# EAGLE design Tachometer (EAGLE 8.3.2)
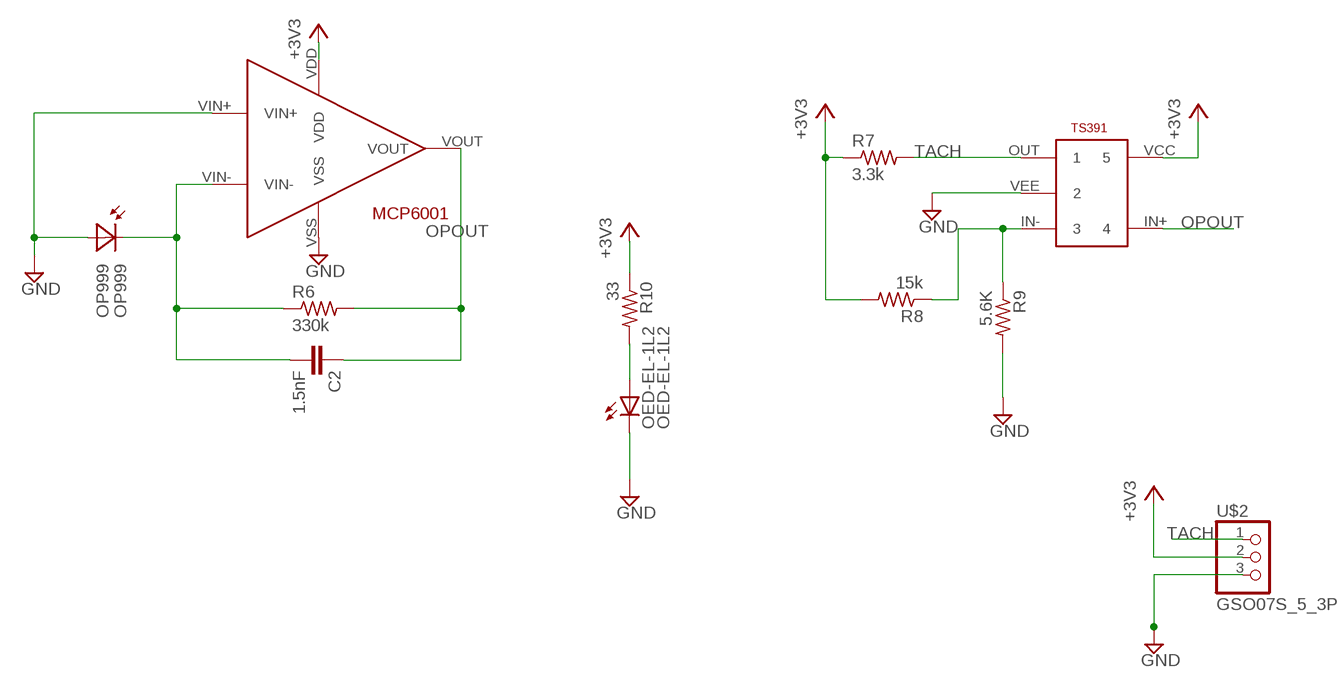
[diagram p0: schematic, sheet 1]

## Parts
C2  1.5nF  UNPCAP  [CAP]
OED-EL-1L2  OED-EL-1L2  [OEL-EL-1L2]
OP999  OP999  [OP999]
R6  330k  R10K  [R10K]
R7  3.3k  R10K  [R10K]
R8  15k  R10K  [R10K]
R9  5.6K  R10K  [R10K]
R10  33  R10K  [R10K]
TS391  TS391  [TS391]
U$1  MCP6001  [MCP6001]
U$2  GSO07S_5_3P  [GSO07S_5_3P]

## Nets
+3V3: R7.1 R8.2 R10.1 TS391.VCC U$1.VDD U$2.2
GND: OED-EL-1L2.2(C) OP999.1(A) R9.2 TS391.VEE U$1.VIN+ U$1.VSS U$2.3
N$1: R8.1 R9.1 TS391.IN-
N$2: C2.2 OP999.2(C) R6.1 U$1.VIN-
N$3: OED-EL-1L2.1(A) R10.2
OPOUT: C2.1 R6.2 TS391.IN+ U$1.VOUT
TACH: R7.2 TS391.OUT U$2.1

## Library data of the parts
C2 = MyLibrary:UNPCAP
OED-EL-1L2 = MyLibrary:OED-EL-1L2
OP999 = MyLibrary:OP999
R6-R10 = MyLibrary:R10K
TS391 = MyLibrary:TS391
U$1 = MyLibrary:MCP6001
U$2 = MyLibrary:GSO07S_5_3P

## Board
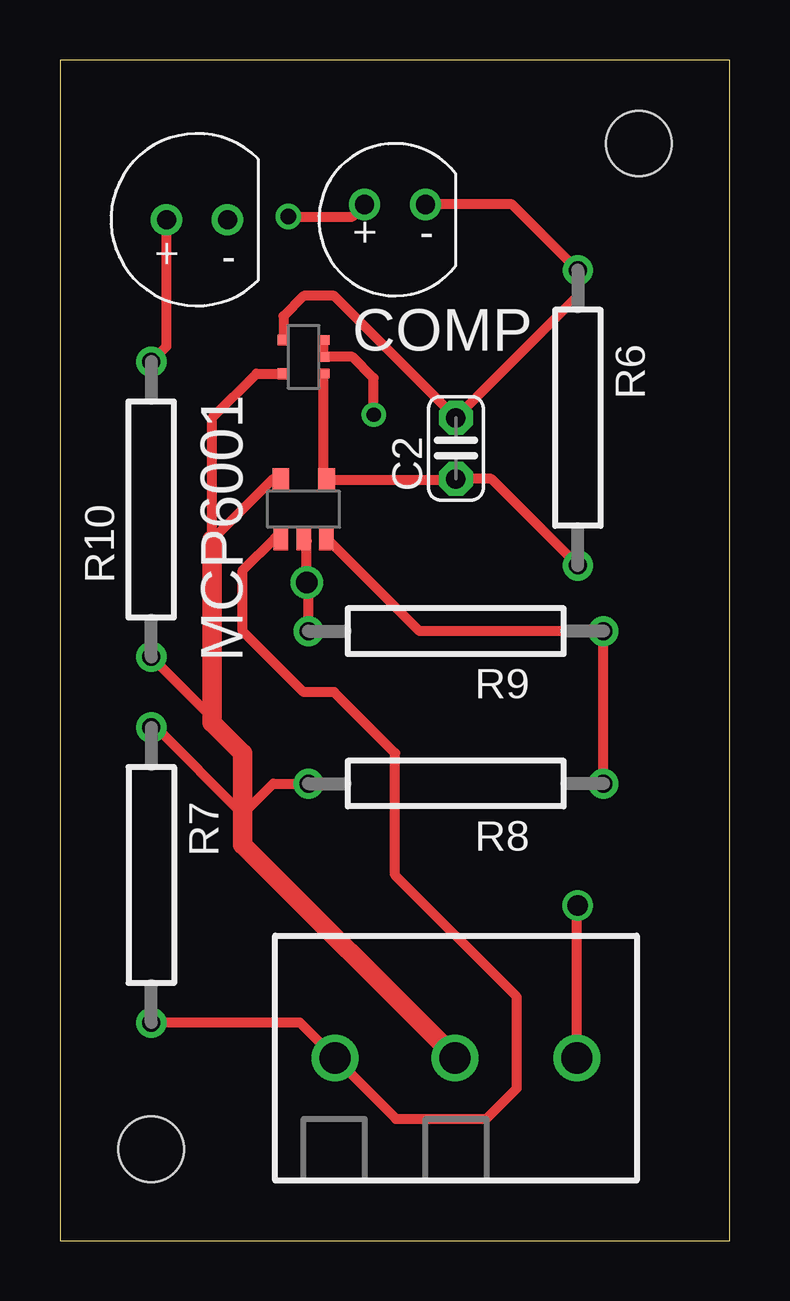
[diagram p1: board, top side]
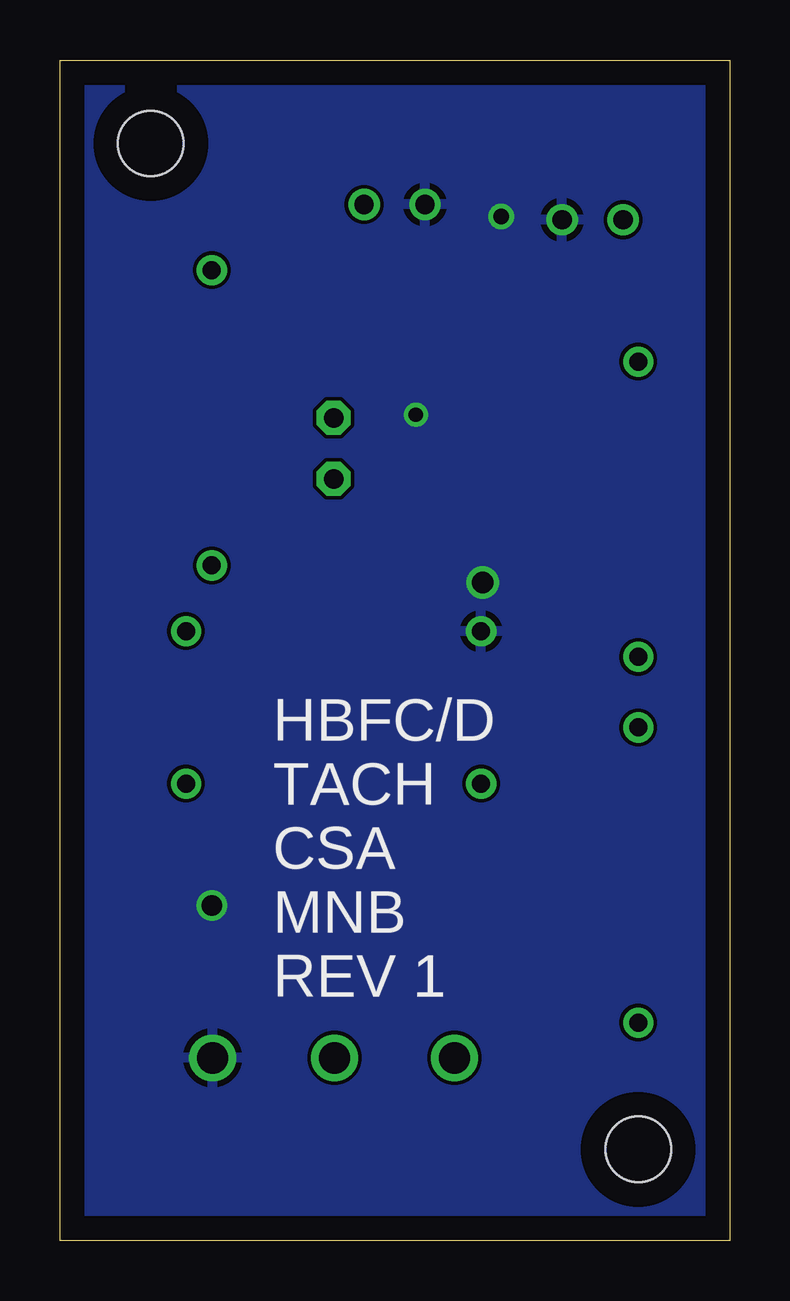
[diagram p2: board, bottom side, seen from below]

Size 27.92 x 49.2 mm. Coordinates in mm from the lower left corner, seen from the top.
Outline: 0,0 27.92,0 27.92,49.2 0,49.2 0,0
Copper layers (1*16): Top 0.035mm / dielectric 1.5mm / Bottom 0.035mm
Design rules "default": minimum track width 6mil, minimum drill 0.35mm, track to track 6mil, track to pad 6mil, pad to pad 6mil, via to via 6mil, smd to smd 6mil, copper to edge 40mil, drill to drill 6mil, minimum pad ring 10mil, minimum via ring 8mil, stop-mask expansion 4mil, vias tented up to drill 0mil, thermal gap 10mil
Holes 2.73 mm at 3.81,3.81 24.13,45.72

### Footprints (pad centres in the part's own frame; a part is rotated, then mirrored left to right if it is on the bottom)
CAP = drill 0.813 pad 1.422 octagon: 1 -1.27,0; 2 1.27,0
OEL-EL-1L2 = drill 0.8: 1 -1.27,0; 2 1.27,0
OP999 = drill 0.8: 1 -1.27,0; 2 1.27,0
R10K = drill 0.75: 1 -6.15,0; 2 6.15,0
TS391 = smd 0.7 x 1: IN+ -0.95,-1.2; VCC 0.95,-1.2 | smd 0.6 x 1: IN- -0.95,1.2; OUT 0.95,1.2; VEE 0,1.2
MCP6001 = smd 0.45 x 0.5: VDD 0.7,-0.838; VIN- -0.7,-0.838 | smd 0.4 x 0.5: VIN+ -0.7,0.838; VOUT 0.7,0.838; VSS 0,0.838
GSO07S_5_3P = drill 1.3: 1 2.58,5.08; 2 7.58,5.08; 3 12.66,5.08

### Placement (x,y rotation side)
C2  16.51,33.02 90 top
OED-EL-1L2  5.71,42.55 0 top
OP999  13.97,43.18 0 top
R6  21.59,34.29 270 top
R7  3.81,15.24 270 top
R8  16.51,19.05 180 top
R9  16.51,25.4 180 top
R10  3.81,30.48 90 top
TS391  10.16,30.48 180 top
U$1  10.16,36.83 270 top
U$2  8.89,2.54 0 top

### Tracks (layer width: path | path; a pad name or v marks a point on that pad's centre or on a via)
+3V3
  Top 0.406: TS391.VCC 9.14,31.75 8.89,31.75 6.35,29.21 6.35,34.29 8.19,36.13 U$1.VDD | 7.62,20.32 7.62,20.52 R10.1 | R8.2 8.89,19.05 7.62,17.78 4.01,21.39 R7.1
  Top 0.813: U$2.2 16.47,7.66 7.62,16.51 7.62,17.78 7.62,20.32 6.35,21.59 6.35,29.21
GND  (via drill 0.6, 0.65, 0.85, 0.9)
  Top 0.406: U$2.3 21.55,13.93 v21.59,13.97 | R9.2 10.36,27.36 v10.29,27.43 10.29,29.15 TS391.VEE | v13.08,34.42 13.08,35.94 12.19,36.83 U$1.VSS U$1.VIN+ | v9.53,42.67 12.19,42.67 OP999.1
  pour Bottom: 0,0 0,49.15 27.81,49.15 27.81,0
N$1
  Top 0.406: TS391.IN- 14.99,25.4 R9.1 R8.1
N$2
  Top 0.406: OP999.2 18.85,43.18 R6.1 21.59,39.37 C2.2 11.43,39.37 10.16,39.37 9.32,38.53 U$1.VIN-
N$3
  Top 0.406: R10.2 4.45,37.27 OED-EL-1L2.1
OPOUT
  Top 0.406: R6.2 17.98,31.75 C2.1 16.44,31.68 TS391.IN+ 11,31.79 U$1.VOUT
TACH
  Top 0.406: R7.2 10,9.09 U$2.1 14.01,5.08 17.78,5.08 19.05,6.35 19.05,10.16 13.97,15.24 13.97,20.32 11.43,22.86 10.16,22.86 7.62,25.4 7.62,27.94 8.96,29.28 TS391.OUT

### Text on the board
tPlace: COMP | MCP6001
bPlace: HBFC/D / TACH / CSA / MNB / REV 1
